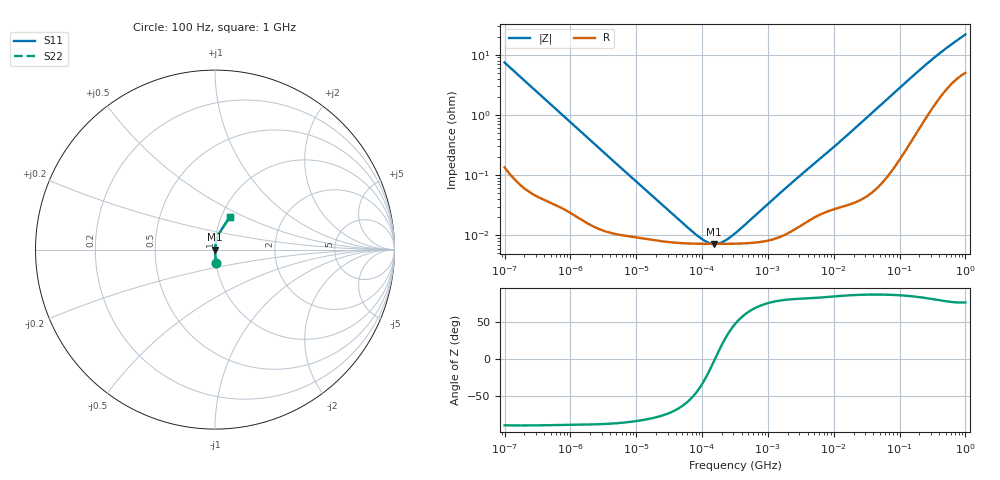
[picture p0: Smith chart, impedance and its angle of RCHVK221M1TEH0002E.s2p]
! RCHVK221M1TEH0002E  S-PARAMETER MODEL  (AEC-Q200 qualified)
! Model Generated by ELNA Corporation (http://www.ty-top.com)
! Version 1.0
! ELNA Control No. 240315
! Copyright (c) 2024 ELNA CO.,LTD. All Rights Reserved.
! Products Name : CONDUCTIVE POLYMER HYBRID ALUMINUM ELECTROLYTIC CAPACITORS
! Characteristics :
!  Capacitance  :  220uF  ,  Rated voltage  :  25V
!  Operating Temp. Range  :  -55 to +125 degC  ,  Endurance  :  4000hr at 125 degC
!  Dimension D  :  8mm  ,  Dimension L  :  10mm
! Frequency Range : 100Hz - 1GHz
! External Node Assignments :
!  1  o---| |---o  2
# MHz S RI R 50
!Freq[MHz].  S11 Real  S11 Imag  S21 Real  S21 Imag  S12 Real  S12 Imag  S22 Real  S22 Imag
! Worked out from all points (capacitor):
!   401 points, 100 Hz to 1 GHz, reference 50 ohm
!   read as one part in series: C = 215 uF near 108 Hz
!   lowest |Z| = 7.19 mohm at 153.1 kHz (marker M1)
!   series resonance near 156.2 kHz, so ESL is about 4.8 nH
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0.0001  0.00678 -0.0735  0.9932 0.0735  0.9932 0.0735  0.00678 -0.0735
0.000113  0.00541 -0.0652  0.9946 0.0652  0.9946 0.0652  0.00541 -0.0652
0.000183  0.00228 -0.0404  0.9977 0.0404  0.9977 0.0404  0.00228 -0.0404
0.000309  0.00102 -0.024  0.999 0.024  0.999 0.024  0.00102 -0.024
0.001488  0.000206 -0.0051  0.9998 0.0051  0.9998 0.0051  0.000206 -0.0051
0.022131  8.09e-05 -0.000351  0.9999 0.000351  0.9999 0.000351  8.09e-05 -0.000351
0.060604  7.32e-05 -0.000113  0.9999 0.000113  0.9999 0.000113  7.32e-05 -0.000113
0.080353  7.24e-05 -7.37e-05  0.9999 7.37e-05  0.9999 7.37e-05  7.24e-05 -7.37e-05
0.090678  7.22e-05 -5.89e-05  0.9999 5.89e-05  0.9999 5.89e-05  7.22e-05 -5.89e-05
0.153109  7.19e-05 -2.03e-06  0.9999 2.03e-06  0.9999 2.03e-06  7.19e-05 -2.03e-06
0.269153  7.22e-05 5.91e-05  0.9999 -5.91e-05  0.9999 -5.91e-05  7.22e-05 5.91e-05
0.291743  7.23e-05 6.89e-05  0.9999 -6.89e-05  0.9999 -6.89e-05  7.23e-05 6.89e-05
0.316228  7.25e-05 7.91e-05  0.9999 -7.91e-05  0.9999 -7.91e-05  7.25e-05 7.91e-05
1.862087  0.000104 0.000599  0.9999 -0.000599  0.9999 -0.000599  0.000104 0.000599
4.704354  0.000191 0.00144  0.9998 -0.00144  0.9998 -0.00144  0.000191 0.00144
13.96368  0.000317 0.00401  0.9997 -0.00401  0.9997 -0.00401  0.000317 0.00401
69.9842  0.00142 0.0197  0.9986 -0.0197  0.9986 -0.0197  0.00142 0.0197
156.6751  0.00573 0.0431  0.9943 -0.0431  0.9943 -0.0431  0.00573 0.0431
323.5937  0.0202 0.0825  0.9798 -0.0825  0.9798 -0.0825  0.0202 0.0825
568.8529  0.0458 0.1264  0.9542 -0.1264  0.9542 -0.1264  0.0458 0.1264
922.5714  0.0781 0.1744  0.9219 -0.1744  0.9219 -0.1744  0.0781 0.1744
1000  0.0845 0.1839  0.9155 -0.1839  0.9155 -0.1839  0.0845 0.1839
